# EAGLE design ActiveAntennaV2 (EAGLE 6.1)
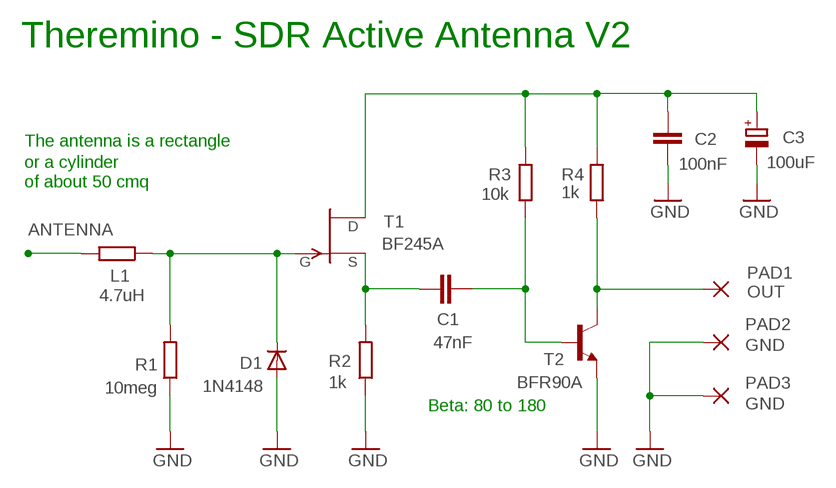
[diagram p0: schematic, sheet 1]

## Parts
C1  47nF  C-EU050-024X044  [C050-024X044]
C2  100nF  C-EU050-024X044  [C050-024X044]
C3  100uF  CPOL-EUE2-5B  [E2-5B]
D1  1N4148  DIODE-DO34-7  [DO34-7]
L1  4.7uH  R-EU_0207/10  [0207/10]
PAD1  OUT  WIREPAD2,54/1,1  [2,54/1,1]
PAD2  GND  WIREPAD2,54/1,1  [2,54/1,1]
PAD3  GND  WIREPAD2,54/1,1  [2,54/1,1]
R1  10meg  R-EU_0204/7  [0204/7]
R2  1k  R-EU_0204/7  [0204/7]
R3  10k  R-EU_0204/7  [0204/7]
R4  1k  R-EU_0204/7  [0204/7]
T1  BF245A  BF245TO92L  [TO92-CBE]
T2  BFR90A  -NPN-BFR90_1  [BFR90]

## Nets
ANTENNA: L1.2
GATE: D1.C L1.1 R1.2 T1.C(G)
GND: C2.2 C3.- D1.A PAD2.1(P) PAD3.1(P) R1.1 R2.1 T2.E
N$1: C1.2 R2.2 T1.B(S)
N$3: C1.1 R3.1 T2.B
N$4: C2.1 C3.+ R3.2 R4.2 T1.E(D)
OUT: PAD1.1(P) R4.1 T2.C

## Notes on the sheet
- Theremino - SDR Active Antenna V2
- The antenna is a rectangle
- or a cylinder
- of about 50 cmq
- Beta: 80 to 180

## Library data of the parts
C1 C2 = 00-LIVIO:C-EU: CAPACITOR, European symbol
C3 = 00-LIVIO:CPOL-EU: POLARIZED CAPACITOR, European symbol
D1 = 00-LIVIO:DIODE-: DIODE
L1 R1-R4 = 00-LIVIO:R-EU_: RESISTOR, European symbol
PAD1-PAD3 = 00-LIVIO:WIREPAD: Wire PAD connect wire on PCB
T1 = 00-LIVIO:BF245: N-Channel Junction FET http://www.onsemi.com/pub/Collateral/BF245A-D.PDF
T2 = 00-LIVIO:*-NPN-: NPN Transistror

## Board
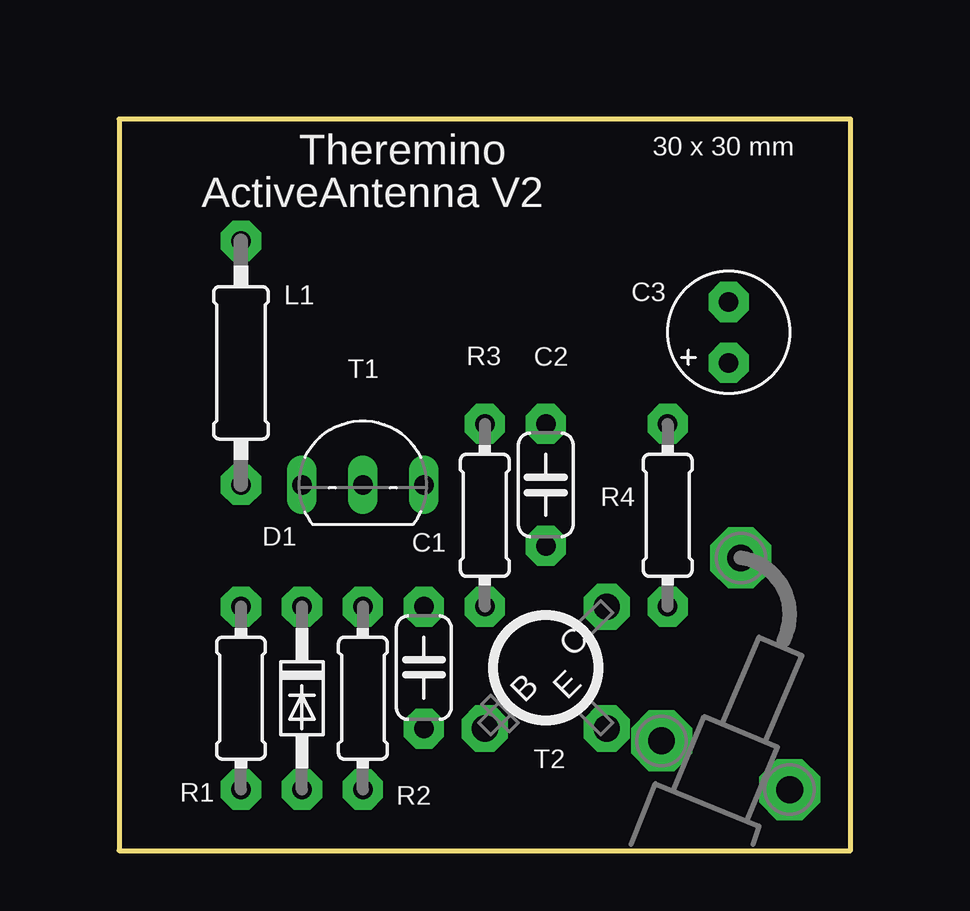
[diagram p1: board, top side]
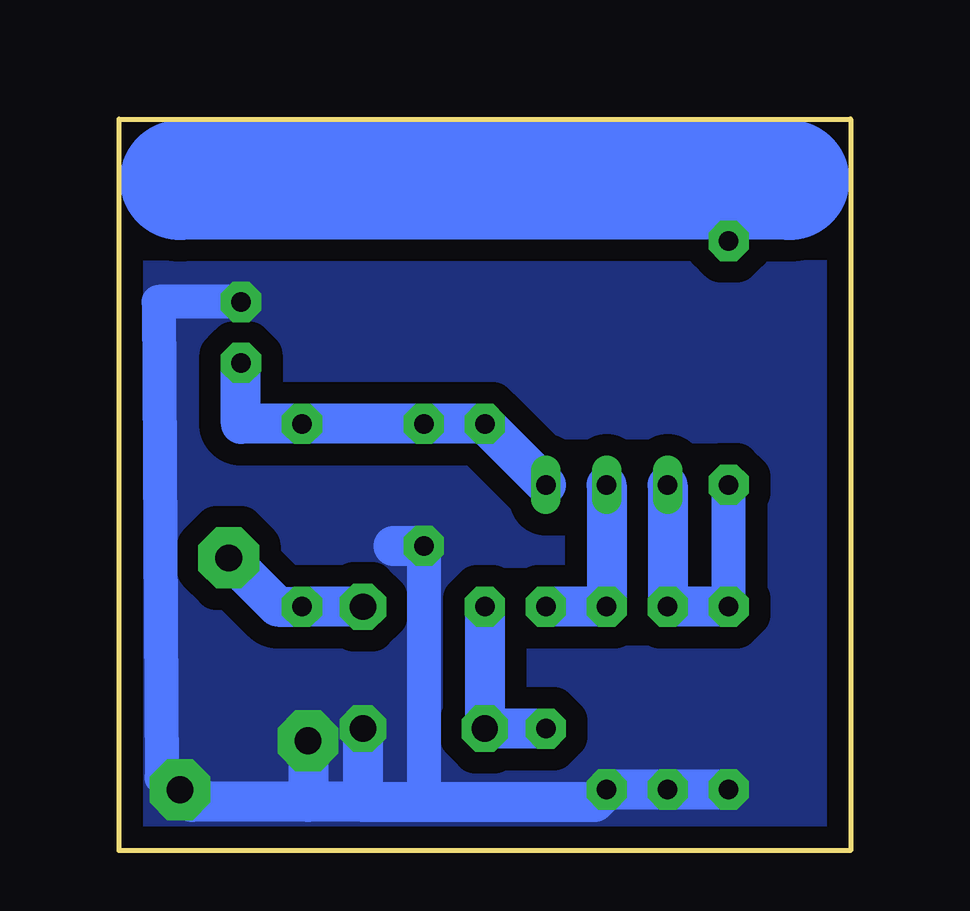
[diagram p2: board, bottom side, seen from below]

Size 30.48 x 30.48 mm. Coordinates in mm from the lower left corner, seen from the top.
Outline: 0,0 30.48,0 30.48,30.48 0,30.48 0,0
Copper layers (1*16): Top 0.035mm / dielectric 1.5mm / Bottom 0.035mm
Design rules: minimum track width 10mil, minimum drill 31mil, track to track 31mil, track to pad 31mil, pad to pad 31mil, via to via 31mil, smd to smd 31mil, copper to edge 31mil, drill to drill 8mil, minimum pad ring 5mil, minimum via ring 8mil, stop-mask expansion 4mil, vias tented up to drill 0mil, thermal gap 47mil

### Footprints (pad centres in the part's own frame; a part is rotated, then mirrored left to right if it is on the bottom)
C050-024X044 = drill 0.813 pad 1.676 octagon: 1 -2.54,0; 2 2.54,0
E2-5B = drill 0.813 pad 1.676 octagon: + -1.27,0; - 1.27,0
DO34-7 = drill 0.813 pad 1.676 octagon: A 3.81,0; C -3.81,0
0207/10 = drill 0.813 pad 1.676 octagon: 1 -5.08,0; 2 5.08,0
2,54/1,1 = drill 1.118 pad 2.54 octagon: 1 0,0
0204/7 = drill 0.813 pad 1.676 octagon: 1 -3.81,0; 2 3.81,0
TO92-CBE = drill 0.813 long: B 0,0; C -2.54,0; E 2.54,0
BFR90 = drill 1.1 pad 1.93 octagon: B -2.54,-2.54; C 2.54,2.54; E 2.54,-2.54

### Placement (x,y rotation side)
C1  12.7,7.62 90 top
C2  17.78,15.24 270 top
C3  25.4,21.59 90 top
D1  7.62,6.35 270 top
L1  5.08,20.32 90 top
PAD1  25.91,12.19 0 top
PAD2  22.61,4.57 0 top
PAD3  27.94,2.54 0 top
R1  5.08,6.35 90 top
R2  10.16,6.35 90 top
R3  15.24,13.97 90 top
R4  22.86,13.97 90 top
T1  10.16,15.24 0 top
T2  17.78,7.62 0 top

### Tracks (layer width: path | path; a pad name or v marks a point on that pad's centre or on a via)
ANTENNA
  Bottom 1.676: L1.2 5.08,27.94
  Bottom 5: 2.54,27.94 5.08,27.94 27.94,27.94
GATE
  Bottom 1.422: R1.2 L1.1
  Bottom 1.676: R1.2 D1.C T1.C
GND
  Bottom 1.422: C2.2 17.78,2.03 | C3.- 28.83,22.86 28.7,3.05 28.19,2.54
  Bottom 1.676: 20.32,2.03 17.78,2.03 10.67,2.03 R2.1 D1.A R1.1 | T2.E 20.32,2.03 | 20.32,2.03 22.61,2.03 | 22.61,2.03 27.43,2.03 PAD3.1 | PAD3.1 27.69,2.54 | 19.05,12.7 C2.2 | PAD2.1 22.61,2.03 | 28.19,2.54 PAD3.1
  pour Bottom (isolate 0.9, rank 6, no thermals): -1,-1 31.48,-1 31.48,31.48 -1,31.48
N$1
  Bottom 1.676: C1.2 R2.2 T1.B
N$3
  Bottom 1.676: C1.1 T2.B R3.1
N$4
  Bottom 1.676: T1.E R3.2 C2.1 R4.2 25.4,17.78 C3.+
OUT
  Bottom 1.676: T2.C R4.1 23.88,10.16 PAD1.1

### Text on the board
tNames: Theremino | 30 x 30 mm | ActiveAntenna V2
